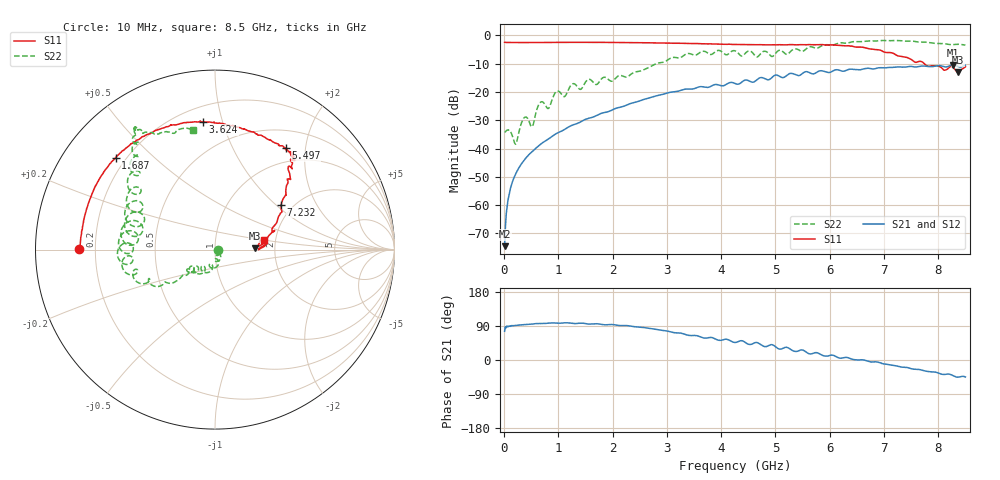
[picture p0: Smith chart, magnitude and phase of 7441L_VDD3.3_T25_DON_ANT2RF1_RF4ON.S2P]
!Agilent Technologies,E5071C,MY46417908,A.11.23
!Date: Mon May 03 19:54:39 2021
!Data & Calibration Information:
!Freq	S11:SOLT2(ON)	S21:SOLT2(ON)	S12:SOLT2(ON)	S22:SOLT2(ON)
!PortZ  Port1:50+j0  Port2:50+j0
!Above PortZ is port z conversion or system Z0 setting when saving the data.
!When reading, reference impedance value at option line is always used.
# Hz S dB R 50
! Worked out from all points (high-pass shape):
!   1601 points, 10 MHz to 8.5 GHz, reference 50 ohm
!   highest |S21| = -10.45 dB at 8.272 GHz (marker M1); lowest = -74.5 dB at 10 MHz (marker M2)
!   |S21| within 3 dB of the highest: 5.498 GHz to 5.658 GHz (159.8 MHz wide, 2.86 % of centre); 5.723 GHz to end of sweep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
!   lowest |S11| = -13.1 dB at 8.367 GHz (marker M3), VSWR 1.57, Z = 78.5 + j1.31 ohm
!   |S11| at or under -10 dB: 7.744 GHz to end of sweep
!   |S22| runs from -38.5 to -1.8 dB; largest |S21 - S12| = 0.008
!   S11 on the Smith chart (normalised r, x): 10 MHz: 0.14, +0.00; 1.687 GHz: 0.16, +0.38; 3.624 GHz: 0.30, +0.87; 5.497 GHz: 0.76, +1.65; 7.232 GHz: 1.74, +1.09; 8.5 GHz: 1.74, +0.21
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1e7  -2.43 179.6  -74.53 75.8  -73.48 78.6  -34.25 -2.6
1.108188e8  -2.49 176.7  -54.55 88.7  -54.71 90.0  -33.84 -37.6
2.169438e8  -2.50 173.6  -48.86 91.4  -48.87 91.5  -38.41 -31.9
3.230688e8  -2.52 170.7  -45.32 92.7  -45.35 92.9  -30.80 -31.6
3.973562e8  -2.51 168.6  -43.46 93.6  -43.44 93.8  -28.87 -61.8
5.194e8  -2.49 165.4  -41.05 94.6  -41.03 94.7  -32.24 -61.3
6.573625e8  -2.49 161.7  -38.71 96.3  -38.73 96.3  -23.92 -66.4
8.1655e8  -2.48 157.7  -36.62 97.4  -36.63 97.4  -25.83 -83.7
9.704312e8  -2.45 153.5  -34.65 97.4  -34.63 97.4  -19.76 -92.8
1.426769e9  -2.44 143.3  -30.38 97.3  -30.39 97.3  -18.85 -119.2
1.554119e9  -2.44 140.1  -29.31 94.8  -29.31 94.9  -15.54 -127.8
1.686775e9  -2.45 137.2  -28.49 95.6  -28.48 95.5  -17.33 -136.9
2.843538e9  -2.67 112.2  -21.18 79.6  -21.20 79.8  -9.75 -145.5
3.623556e9  -2.91 95.2  -18.10 60.6  -18.12 60.4  -5.86 -165.0
4.255e9  -3.20 77.8  -16.98 46.4  -16.98 45.8  -5.42 173.0
5.496662e9  -3.23 55.1  -13.47 26.5  -13.43 26.1  -5.63 143.1
5.671769e9  -3.29 51.8  -13.55 16.5  -13.52 16.0  -4.05 136.0
7.088538e9  -6.04 37.4  -11.32 -12.4  -11.32 -12.9  -1.88 123.4
7.231806e9  -7.01 34.2  -11.18 -15.7  -11.14 -16.1  -1.78 122.9
8.271831e9  -11.30 6.9  -10.45 -41.4  -10.47 -41.4  -3.25 109.0
8.367344e9  -13.06 2.0  -11.04 -45.3  -11.07 -45.4  -3.11 105.4
8.5e9  -11.07 11.5  -10.52 -44.9  -10.54 -44.8  -3.40 100.4
